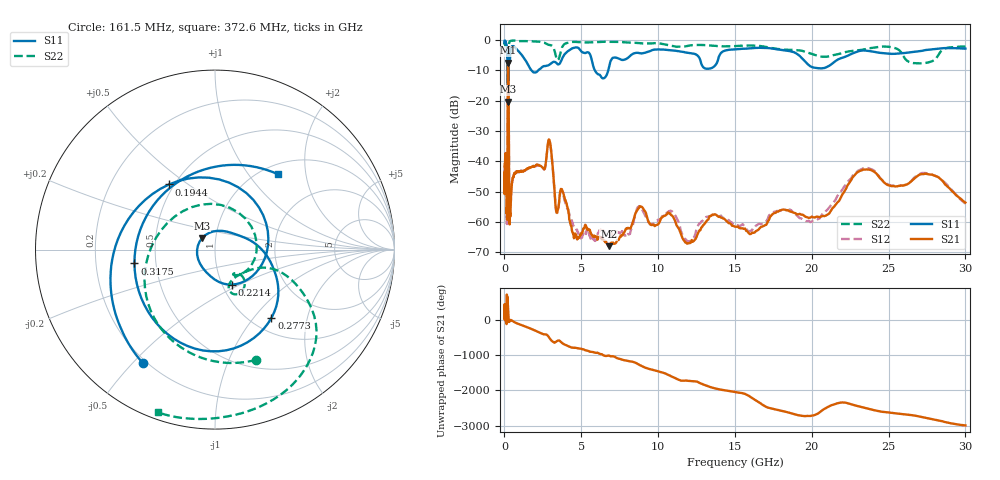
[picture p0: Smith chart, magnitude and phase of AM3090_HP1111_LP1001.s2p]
! Date/Time: Thu, Feb 28, 2019 2:10 PM
! Network Analyzer: Agilent Technologies E8364B Rev: A.07.50.67
! Sweep from 0.010 to 30.000 GHz, 1601 Points, Sweep Type: LOG
! Power Supply: 5.023 V, 0.002 A
# Hz S DB R 50
!freq MagS11 AngS11 MagS21 AngS21 MagS12 AngS12 MagS22 AngS22
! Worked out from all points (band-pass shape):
!   1601 points, 10 MHz to 30 GHz, reference 50 ohm
!   highest |S21| = -7.46 dB at 238.7 MHz (marker M1); lowest = -68.1 dB at 6.787 GHz (marker M2)
!   |S21| within 3 dB of the highest: 215.2 MHz to 263 MHz (47.83 MHz wide, 20 % of centre)
!   lowest |S11| = -20.3 dB at 237.5 MHz (marker M3), VSWR 1.21, Z = 43 + j5.56 ohm
!   |S11| at or under -10 dB: 206.9 MHz to 261.3 MHz (54.34 MHz wide, 23.2 % of centre); 1.763 GHz to 2.199 GHz (435.8 MHz wide, 22 % of centre); 5.884 GHz to 6.756 GHz (871.6 MHz wide, 13.8 % of centre)
!   |S22| runs from -15.4 to -0.1 dB; largest |S21 - S12| = 0.011
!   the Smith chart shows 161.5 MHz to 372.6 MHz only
!   S11 on the Smith chart (normalised r, x): 161.5 MHz: 0.19, -0.53; 194.4 MHz: 0.47, +0.42; 221.4 MHz: 1.11, -0.45; 277.3 MHz: 1.23, -1.24; 317.5 MHz: 0.38, -0.07; 372.6 MHz: 1.17, +1.40
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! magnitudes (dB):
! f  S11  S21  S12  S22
! 10 MHz  -0.3  -46.3  -45.4  -0.7
! 38.04 MHz  -0.2  -40.8  -41.1  -1.2
! 105.1 MHz  -1.0  -40.3  -39.8  -3.3
! 144.7 MHz  -1.7  -57.1  -56.2  -3.4
! 161.5 MHz  -2.5  -56.5  -58.8  -3.7
! 181.3 MHz  -4.5  -59.4  -58.6  -6.7
! 194.4 MHz  -7.0  -39.0  -39.3  -11.8
! 221.4 MHz  -13.3  -8.6  -8.5  -14.7
! 237.5 MHz  -20.3  -7.5  -7.4  -11.1
! 238.7 MHz  -20.3  -7.5  -7.4  -11.2
! 277.3 MHz  -6.1  -21.0  -21.1  -6.2
! 317.5 MHz  -6.8  -57.4  -57.6  -0.8
! 372.6 MHz  -5.2  -58.4  -57.8  -0.3
! 550.5 MHz  -2.0  -45.6  -45.8  -0.2
! 2.084 GHz  -10.6  -41.2  -41.5  -0.5
! 2.928 GHz  -8.1  -33.0  -32.9  -1.6
! 3.402 GHz  -7.7  -56.9  -57.1  -6.3
! 6.787 GHz  -9.3  -68.1  -64.7  -0.6
! 7.926 GHz  -6.2  -62.2  -65.1  -0.8
! 20 GHz  -8.9  -58.3  -59.9  -4.6
! 23.36 GHz  -3.4  -42.8  -42.3  -3.1
! 30 GHz  -2.8  -53.7  -54.0  -2.2
